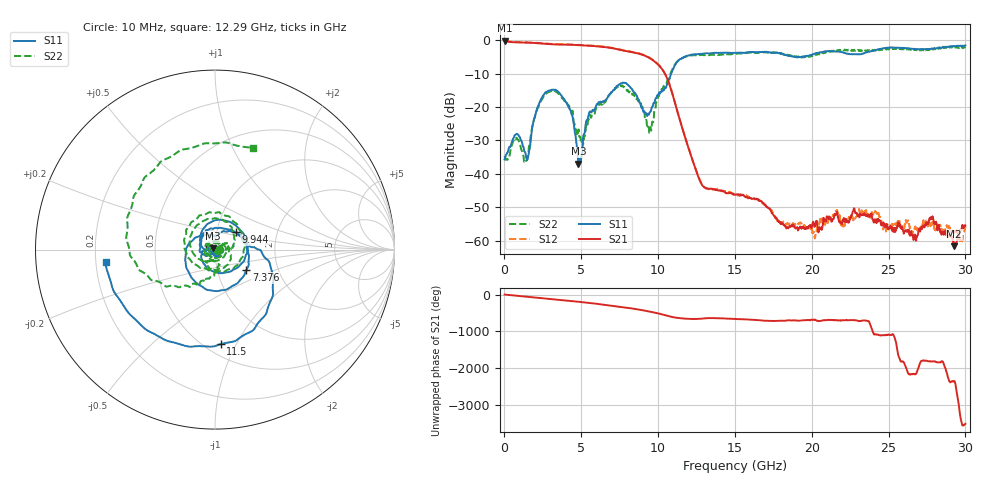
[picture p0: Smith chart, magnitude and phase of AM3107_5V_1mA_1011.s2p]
# Hz S DB R 50.0
!freq dBS11 angS11 dBS21 angS21 dBS12 angS12 dBS22 angS22
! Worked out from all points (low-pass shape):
!   1601 points, 10 MHz to 30 GHz, reference 50 ohm
!   highest |S21| = -0.12 dB at 10 MHz (marker M1); lowest = -61.7 dB at 29.27 GHz (marker M2)
!   |S21| within 3 dB of the highest: start of sweep to 7.765 GHz
!   lowest |S11| = -37.0 dB at 4.808 GHz (marker M3), VSWR 1.03, Z = 48.9 + j0.798 ohm
!   |S11| at or under -10 dB: start of sweep to 10.85 GHz
!   |S22| runs from -36.4 to -1.8 dB; largest |S21 - S12| = 0.012
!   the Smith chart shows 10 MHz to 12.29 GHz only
!   S11 on the Smith chart (normalised r, x): 10 MHz: 1.01, -0.03; 7.376 GHz: 1.38, -0.32; 9.944 GHz: 1.23, +0.24; 11.5 GHz: 0.59, -0.87; 12.29 GHz: 0.24, -0.05
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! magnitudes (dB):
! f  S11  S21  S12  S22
! 10 MHz  -35.7  -0.1  -0.1  -34.6
! 797.2 MHz  -28.1  -0.6  -0.5  -29.3
! 1.416 GHz  -35.1  -0.7  -0.6  -36.1
! 2.166 GHz  -20.0  -0.9  -0.8  -20.4
! 3.196 GHz  -14.8  -1.2  -1.1  -15.2
! 4.302 GHz  -21.0  -1.4  -1.3  -20.2
! 4.808 GHz  -37.0  -1.4  -1.3  -26.9
! 5.015 GHz  -34.7  -1.5  -1.4  -30.7
! 5.483 GHz  -22.4  -1.6  -1.5  -23.8
! 7.376 GHz  -13.6  -2.7  -2.6  -14.1
! 9.419 GHz  -22.1  -5.3  -5.2  -27.7
! 9.944 GHz  -16.5  -7.0  -6.9  -18.2
! 10.02 GHz  -16.3  -7.4  -7.2  -16.8
! 11.5 GHz  -5.6  -25.2  -25.1  -5.7
! 12.29 GHz  -4.2  -36.6  -36.6  -4.4
! 15.01 GHz  -3.7  -46.2  -46.3  -4.0
! 20.01 GHz  -4.3  -55.8  -57.3  -4.7
! 23.16 GHz  -4.2  -52.1  -51.8  -3.1
! 25.01 GHz  -2.2  -56.4  -56.6  -2.7
! 27.77 GHz  -2.6  -53.4  -55.7  -2.9
! 29.27 GHz  -1.7  -61.7  -57.7  -1.9
! 30 GHz  -1.5  -55.5  -55.9  -1.9
